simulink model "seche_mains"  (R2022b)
settings: Solver=VariableStepAuto  StartTime=0.0  StopTime=inf  RelTol=1e-3
libraries: realtime_pacer_lib x1

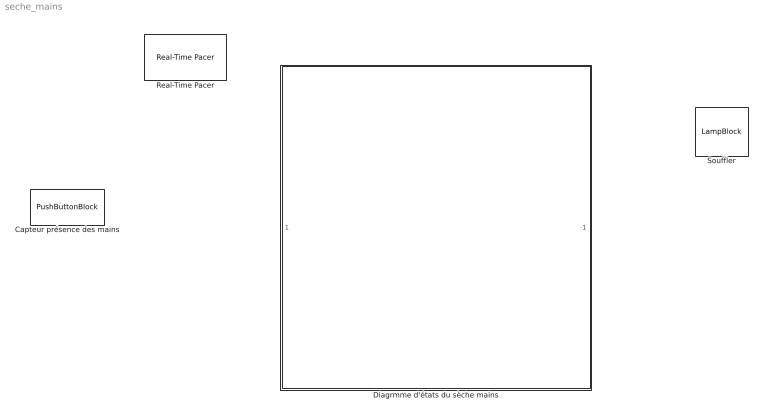
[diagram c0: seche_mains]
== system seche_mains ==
  Capteur présence des mains : PushButtonBlock
  Diagrmme d'états du sèche mains : Stateflow chart  TreatAsAtomicUnit=on
  Real-Time Pacer : realtime_pacer_lib/Real-Time Pacer  simTimePerRealTime=1
  Souffler : LampBlock  LabelPosition=Hide

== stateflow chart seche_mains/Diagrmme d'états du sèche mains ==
  state ?
  state ?
  (default) -> ?
